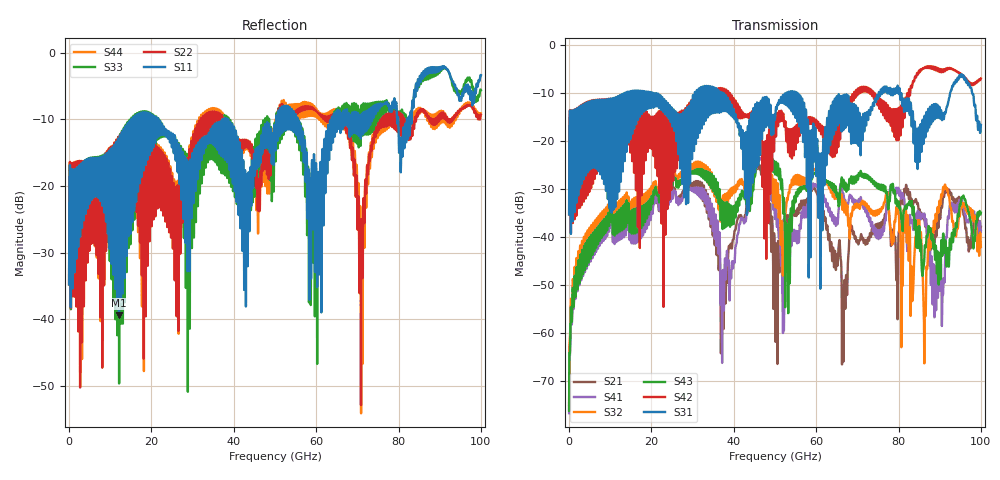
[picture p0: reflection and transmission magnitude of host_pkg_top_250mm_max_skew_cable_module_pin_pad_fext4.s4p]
# Hz S RI R 50
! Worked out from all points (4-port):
!   10000 points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, 10 MHz to 100 GHz, reference 50 ohm
!   strongest paths, dB at 10 MHz, 25.01 GHz, 50.01 GHz, 75.01 GHz, 100 GHz:
!     S31: -35.3, -14.5, -15.3, -11.2, -16.7
!     S42: -35.3, -14.4, -15.0, -11.9, -7.0
!     S43: -76.2, -28.7, -26.8, -29.2, -35.0
!     S32: -75.1, -27.6, -33.6, -34.4, -42.1
!     S41: -76.7, -31.5, -36.3, -39.2, -38.8
!     S21: -75.9, -31.2, -45.6, -38.4, -37.9
!   lowest |S11| = -39.4 dB at 12.13 GHz (marker M1), VSWR 1.02, Z = 50.9 - j0.651 ohm
!   |S11| at or under -10 dB: start of sweep to 15.11 GHz; 21.62 GHz to 37.23 GHz (15.61 GHz wide, 53 % of centre); 38.64 GHz to 50.3 GHz (11.66 GHz wide, 26.2 % of centre)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
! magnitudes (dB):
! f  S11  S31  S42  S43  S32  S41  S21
! 10 MHz  -34.8  -35.3  -35.3  -76.2  -75.1  -76.7  -75.9
! 12.13 GHz  -39.4  -27.6  -18.5  -34.8  -32.6  -36.0  -34.7
! 46.58 GHz  -14.4  -11.7  -21.4  -21.0  -21.6  -23.9  -26.6
! 51.9 GHz  -10.2  -10.6  -14.7  -31.9  -47.9  -57.3  -37.2
! 65.65 GHz  -8.7  -14.5  -16.3  -33.3  -31.3  -31.7  -40.7
! 70.88 GHz  -12.3  -17.2  -9.9  -26.5  -32.9  -31.8  -39.5
! 100 GHz  -3.4  -16.7  -7.0  -35.0  -42.1  -38.8  -37.9
